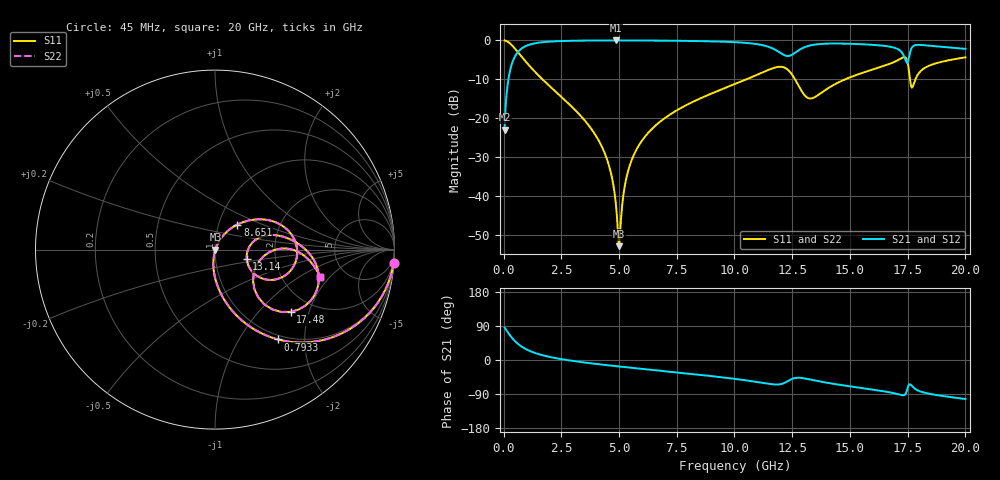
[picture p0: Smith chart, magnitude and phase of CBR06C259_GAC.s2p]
! S-parameter model data by Modelithics Inc.  support@modelithics.com 813-866-6335  Tampa FL USA
! S-Parameter data specifications:
! Substrate: 20-mil Rogers 4350B, substrate thickness, H=0.508mm, Dielectric constant, Er=3.75
! PCB Mounting Pad Footprint: Pad width, PadW=0.85mm , Pad length, PadL=0.64mm , Pad gap, PadG (edge-to-edge)=0.62mm , Reference planes=1.9mm apart
#  GHz  S  MA  R 50
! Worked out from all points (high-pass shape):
!   801 points, 45 MHz to 20 GHz, reference 50 ohm
!   highest |S21| = -0.02 dB at 4.884 GHz (marker M1); lowest = -22.9 dB at 45 MHz (marker M2)
!   |S21| within 3 dB of the highest: 618.2 MHz to 11.94 GHz (11.32 GHz wide, 180 % of centre); 12.66 GHz to 17.24 GHz (4.574 GHz wide, 30.6 % of centre)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
!   lowest |S11| = -52.9 dB at 5.009 GHz (marker M3), VSWR 1.00, Z = 50.2 - j0.0268 ohm
!   |S11| at or under -10 dB: 1.683 GHz to 10.52 GHz (8.837 GHz wide, 145 % of centre); 12.62 GHz to 14.79 GHz (2.174 GHz wide, 15.9 % of centre); 17.6 GHz to 17.84 GHz (235.2 MHz wide, 1.33 % of centre)
!   |S22| runs from -52.9 to 0.0 dB; largest |S21 - S12| = 0
!   S11 on the Smith chart (normalised r, x): 45 MHz: 1, -27; 793.3 MHz: 0.93, -1.49; 8.651 GHz: 1.23, +0.36; 13.14 GHz: 1.42, -0.16; 17.48 GHz: 1.54, -1.52; 20 GHz: 3.26, -1.57
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0.045  0.9974 -4.3  0.0715 85.7  0.0715 85.7  0.9974 -4.3
0.319381  0.8904 -28.1  0.4547 61.8  0.4547 61.8  0.8904 -28.1
0.793312  0.6111 -55.0  0.7905 34.9  0.7905 34.9  0.6111 -55.0
1.666344  0.3198 -76.8  0.946 12.9  0.946 12.9  0.3198 -76.8
3.387462  0.1035 -94.6  0.9926 -5.7  0.9926 -5.7  0.1035 -94.6
4.4351  0.03227 -99.6  0.9972 -13.3  0.9972 -13.3  0.03227 -99.6
4.884087  0.006799 -87.4  0.9975 -16.3  0.9975 -16.3  0.006799 -87.4
5.008806  0.002272 -6.7  0.9975 -17.2  0.9975 -17.2  0.002272 -6.7
5.258244  0.01397 61.7  0.9973 -18.8  0.9973 -18.8  0.01397 61.7
5.532625  0.02818 64.6  0.9969 -20.5  0.9969 -20.5  0.02818 64.6
6.704981  0.08668 60.3  0.993 -27.8  0.993 -27.8  0.08668 60.3
8.650594  0.1871 48.2  0.9766 -40.1  0.9766 -40.1  0.1871 48.2
10.0225  0.2754 37.4  0.9478 -49.9  0.9478 -49.9  0.2754 37.4
12.06789  0.456 -7.2  0.6676 -62.7  0.6676 -62.7  0.456 -7.2
13.14047  0.1849 -16.9  0.839 -49.8  0.839 -49.8  0.1849 -16.9
13.36496  0.1806 -3.5  0.8718 -52.6  0.8718 -52.6  0.1806 -3.5
16.68248  0.494 1.1  0.8347 -84.9  0.8347 -84.9  0.494 1.1
17.28113  0.6012 -15.8  0.6776 -93.2  0.6776 -93.2  0.6012 -15.8
17.48068  0.5453 -39.5  0.5112 -77.5  0.5112 -77.5  0.5453 -39.5
17.70518  0.2497 -18.1  0.825 -69.9  0.825 -69.9  0.2497 -18.1
17.95461  0.3688 0.9  0.8763 -80.7  0.8763 -80.7  0.3688 0.9
20  0.6057 -14.6  0.7777 -103.0  0.7777 -103.0  0.6057 -14.6
